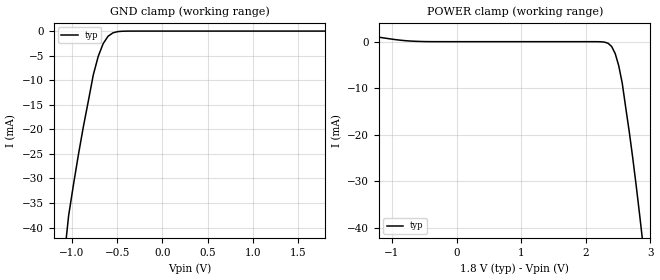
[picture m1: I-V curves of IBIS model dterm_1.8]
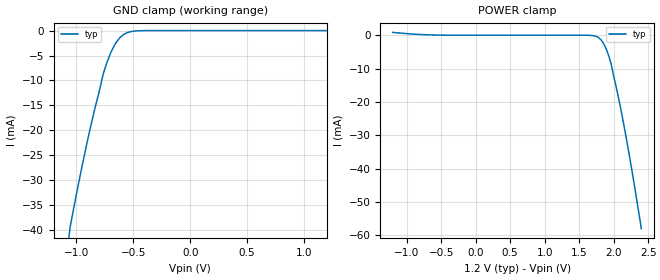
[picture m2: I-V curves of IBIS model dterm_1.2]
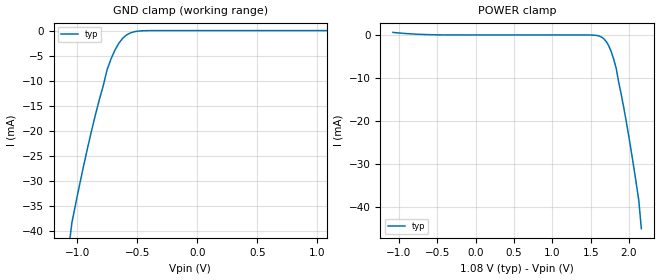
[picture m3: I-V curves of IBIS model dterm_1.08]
|Texas Instruments Incorporated
|tmuxl27518, 6 Data Lane 2:1 Switch
[IBIS Ver]   4.1
[File name]   tmuxl27518.ibs
[Date]   05/21/26
[File Rev]   1.0
[Source]
| Texas Instruments Incorporated.
| ASC-INT-MPD
| 12500 TI Blvd
| Dallas, TX - 75243
[Notes]   Revision History:
| Rev 1.0: 05/21/26
| - Initial version of the model
| - Model generated from simulations in SPECTRE
| - C_comp although listed in numerical order of value are
|   obtained from varying PVT conditions. For PVT conditions for
|   each specific value refer the buffer description under
|   respective [Model]. IBIS model user is responsible for using
|   appropriate C_comp to simulate for Signal Integrity.
[Disclaimer]
| This model is designed as an aid for customers of Texas Instruments.
| TI and its licensors and suppliers make no warranties, either expressed
| or implied, with respect to this  model, including the warranties of
| merchantability or fitness for a particular purpose. The model is
| provided solely on an "as is" basis. The entire risk as to its quality
| and performance is with the customer.
| This model is subject to change without notice. Texas Instruments
| Incorporated is not responsible for updating this model.
[Copyright]
(C) Copyright 2026 Texas Instruments Incorporated.All rights reserved.
|  Component TMUXL27518RTW 23-pin - RTW package
|  Part # TMUXL27518RTW
[Component]   TMUXL27518RTW
[Manufacturer]  TI
[Package]
|   typ   min   max
R_pkg   0.15   NA   NA
L_pkg   2nH   NA   NA
C_pkg   0.37pF   NA   NA
[Pin]   signal_name   model_name
   1   COM1   dterm
   2   GND   gnd
   3   COM2   dterm
   4   COM3   dterm
   5   VCC   power
   6   COM4   dterm
   7   COM5   dterm
   8   NO1   sterm
   9   COM6   dterm
   10   NO2   sterm
   11   IN2   inbuf
   12   NO3   sterm
   13   NO6   sterm
   14   NO4   sterm
   15   NO5   sterm
   16   NC5   sterm
   17   ENB   inbuf
   18   NC4   sterm
   19   NC6   sterm
   20   NC3   sterm
   21   IN1   inbuf
   22   NC2   sterm
   23   NC1   sterm
[Series Switch Groups]
On 1 /
On 2 /
Off 1 /
[Series Pin Mapping]  pin_2 model_name function_table_group
   1  23   switch_1.8   1
   3  22   switch_1.8   1
   4  20   switch_1.8   1
   6  18   switch_1.8   1
   7  16   switch_1.8   1
   9  19   switch_1.8   1
   1   8   switch_1.8   2
   3  10   switch_1.8   2
   4  12   switch_1.8   2
   6  14   switch_1.8   2
   7  15   switch_1.8   2
   9  13   switch_1.8   2
|   1  23   switch_1.2   1
|   3  22   switch_1.2   1
|   4  20   switch_1.2   1
|   6  18   switch_1.2   1
|   7  16   switch_1.2   1
|   9  19   switch_1.2   1
|   1   8   switch_1.2   2
|   3  10   switch_1.2   2
|   4  12   switch_1.2   2
|   6  14   switch_1.2   2
|   7  15   switch_1.2   2
|   9  13   switch_1.2   2
|   1  23   switch_1.08   1
|   3  22   switch_1.08   1
|   4  20   switch_1.08   1
|   6  18   switch_1.08   1
|   7  16   switch_1.08   1
|   9  19   switch_1.08   1
|   1   8   switch_1.08   2
|   3  10   switch_1.08   2
|   4  12   switch_1.08   2
|   6  14   switch_1.08   2
|   7  15   switch_1.08   2
|   9  13   switch_1.08   2
|   1  23   switch_1.98   1
|   3  22   switch_1.98   1
|   4  20   switch_1.98   1
|   6  18   switch_1.98   1
|   7  16   switch_1.98   1
|   9  19   switch_1.98   1
|   1   8   switch_1.98   2
|   3  10   switch_1.98   2
|   4  12   switch_1.98   2
|   6  14   switch_1.98   2
|   7  15   switch_1.98   2
|   9  13   switch_1.98   2
[Model Selector] dterm
dterm_1.8 Use for operation at 1V
dterm_1.2 Use for operation at 1V
dterm_1.08 Use for operation at 1V
dterm_1.98 Use for operation at 1V
[Model Selector] sterm
sterm_1.8 Use for operation at 1V
sterm_1.2 Use for operation at 1V
sterm_1.08 Use for operation at 1V
sterm_1.98 Use for operation at 1V
[Model Selector] inbuf
inbuf_1.8 Use for operation at 1V
inbuf_1.2 Use for operation at 1V
inbuf_1.08 Use for operation at 1V
inbuf_1.98 Use for operation at 1V
| switch_1.8
[Model]   switch_1.8
Model_type   Series_switch
|   typ   min   max
C_comp   4.014581e-12   NA   NA
[Voltage Range]   1.8   NA   NA
[Power Clamp Reference]   1.8   NA   NA
[Temperature Range]   27   NA   NA
[On]
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[Off]
|   typ   min   max
[R Series]   10G   NA   NA
| switch_1.2
[Model]   switch_1.2
Model_type   Series_switch
|   typ   min   max
C_comp   1.598234e-12   NA   NA
[Voltage Range]   1.2   NA   NA
[Power Clamp Reference]   1.2   NA   NA
[Temperature Range]   27   NA   NA
[On]
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[Off]
|   typ   min   max
[R Series]   10G   NA   NA
| switch_1.08
[Model]   switch_1.08
Model_type   Series_switch
|   typ   min   max
C_comp   1.598234e-12   NA   NA
[Voltage Range]   1.08   NA   NA
[Power Clamp Reference]   1.08   NA   NA
[Temperature Range]   27   NA   NA
[On]
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[Off]
|   typ   min   max
[R Series]   10G   NA   NA
| switch_1.98
[Model]   switch_1.98
Model_type   Series_switch
|   typ   min   max
C_comp   4.014581e-12   NA   NA
[Voltage Range]   1.98   NA   NA
[Power Clamp Reference]   1.98   NA   NA
[Temperature Range]   27   NA   NA
[On]
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[Off]
|   typ   min   max
[R Series]   10G   NA   NA
| Models and submodels in the file (16): dterm_1.8 (Terminator), dterm_1.2 (Terminator), dterm_1.08 (Terminator), dterm_1.98 (Terminator), switch_1.8 (Series_switch), switch_1.2 (Series_switch), switch_1.08 (Series_switch), switch_1.98 (Series_switch), sterm_1.8 (Terminator), sterm_1.2 (Terminator), sterm_1.08 (Terminator), sterm_1.98 (Terminator), inbuf_1.8 (Input), inbuf_1.2 (Input), inbuf_1.08 (Input), inbuf_1.98 (Input)
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| dterm_1.8
[Model]   dterm_1.8
Model_type   Terminator
|   typ   min   max
C_comp   4.014581e-12   NA   NA
[Voltage Range]   1.8   NA   NA
[Temperature Range]   27   NA   NA
[Power Clamp Reference]   1.8   NA   NA
[GND Clamp Reference]   0   NA   NA
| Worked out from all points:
|   GND clamp passes 1 mA (typ) near -0.60 V on its own axis
|   POWER clamp passes 1 mA (typ) near -1.22 V on its own axis
[GND Clamp]
|   Voltage   I(typ)   I(min)   I(max)
-3.6V     -9.241kA   NA         NA
-1.091V   -47.13mA   NA         NA
-1.036V   -37.57mA   NA         NA
-927.3mV  -25.07mA   NA         NA
-872.7mV  -19.39mA   NA         NA
-763.6mV  -8.906mA   NA         NA
-709.1mV  -5.142mA   NA         NA
-654.5mV  -2.546mA   NA         NA
-600mV    -1.043mA   NA         NA
-545.5mV  -351.2uA   NA         NA
-436.4mV  -24.75uA   NA         NA
1.8V      283.7pA    NA         NA
[POWER Clamp]
|   Voltage   I(typ)   I(min)   I(max)
-1.8V     2.361mA    NA         NA
-654.5mV  94.31uA    NA         NA
2.182V    -5.252uA   NA         NA
2.345V    -351.2uA   NA         NA
2.4V      -1.043mA   NA         NA
2.455V    -2.546mA   NA         NA
2.509V    -5.142mA   NA         NA
2.564V    -8.906mA   NA         NA
2.727V    -25.07mA   NA         NA
2.836V    -37.57mA   NA         NA
2.891V    -44.28mA   NA         NA
3.6V      -143.9mA   NA         NA
| dterm_1.2
[Model]   dterm_1.2
Model_type   Terminator
|   typ   min   max
C_comp   4.014581e-12   NA   NA
[Voltage Range]   1.2   NA   NA
[Temperature Range]   27   NA   NA
[Power Clamp Reference]   1.2   NA   NA
[GND Clamp Reference]   0   NA   NA
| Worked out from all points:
|   GND clamp passes 1 mA (typ) near -0.60 V on its own axis
[GND Clamp]
|   Voltage   I(typ)   I(min)   I(max)
-2.4V     -249.7mA   NA         NA
-1.091V   -46.55mA   NA         NA
-1.055V   -39.43mA   NA         NA
-981.8mV  -30.82mA   NA         NA
-909.1mV  -22.81mA   NA         NA
-763.6mV  -8.671mA   NA         NA
-690.9mV  -4.086mA   NA         NA
-654.5mV  -2.521mA   NA         NA
-581.8mV  -737.9uA   NA         NA
-509.1mV  -154.8uA   NA         NA
-400mV    -8.942uA   NA         NA
1.2V      184.3pA    NA         NA
[POWER Clamp]
|   Voltage   I(typ)   I(min)   I(max)
-1.2V     844.1uA    NA         NA
-509.1mV  26.69uA    NA         NA
1.636V    -24.74uA   NA         NA
1.782V    -737.9uA   NA         NA
1.855V    -2.521mA   NA         NA
1.891V    -4.086mA   NA         NA
1.927V    -6.142mA   NA         NA
1.964V    -8.671mA   NA         NA
2.073V    -19.08mA   NA         NA
2.182V    -30.82mA   NA         NA
2.291V    -43.93mA   NA         NA
2.4V      -57.99mA   NA         NA
| dterm_1.08
[Model]   dterm_1.08
Model_type   Terminator
|   typ   min   max
C_comp   4.014581e-12   NA   NA
[Voltage Range]   1.08   NA   NA
[Temperature Range]   27   NA   NA
[Power Clamp Reference]   1.08   NA   NA
[GND Clamp Reference]   0   NA   NA
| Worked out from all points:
|   GND clamp passes 1 mA (typ) near -0.60 V on its own axis
[GND Clamp]
|   Voltage   I(typ)   I(min)   I(max)
-2.16V    -205.3mA   NA         NA
-1.08V    -44.98mA   NA         NA
-1.047V   -38.47mA   NA         NA
-916.4mV  -23.51mA   NA         NA
-850.9mV  -16.88mA   NA         NA
-752.7mV  -7.794mA   NA         NA
-687.3mV  -3.886mA   NA         NA
-654.5mV  -2.511mA   NA         NA
-621.8mV  -1.513mA   NA         NA
-556.4mV  -441.3uA   NA         NA
-392.7mV  -7.24uA    NA         NA
1.08V     165.6pA    NA         NA
[POWER Clamp]
|   Voltage   I(typ)   I(min)   I(max)
-1.08V    590.9uA    NA         NA
-490.9mV  21.51uA    NA         NA
1.505V    -18.36uA   NA         NA
1.604V    -216.2uA   NA         NA
1.669V    -846.4uA   NA         NA
1.735V    -2.511mA   NA         NA
1.767V    -3.886mA   NA         NA
1.833V    -7.794mA   NA         NA
1.964V    -20.11mA   NA         NA
2.062V    -30.75mA   NA         NA
2.127V    -38.47mA   NA         NA
2.16V     -44.98mA   NA         NA
